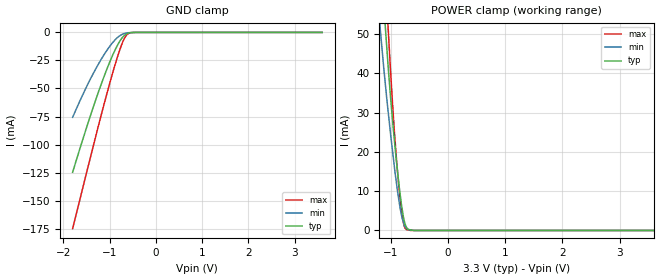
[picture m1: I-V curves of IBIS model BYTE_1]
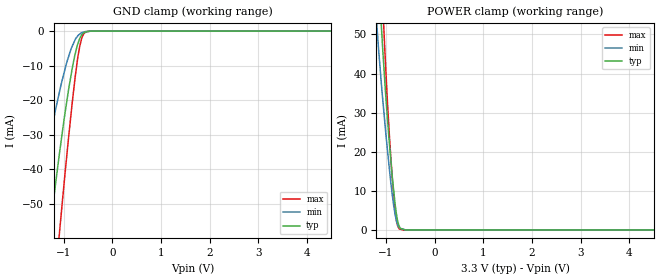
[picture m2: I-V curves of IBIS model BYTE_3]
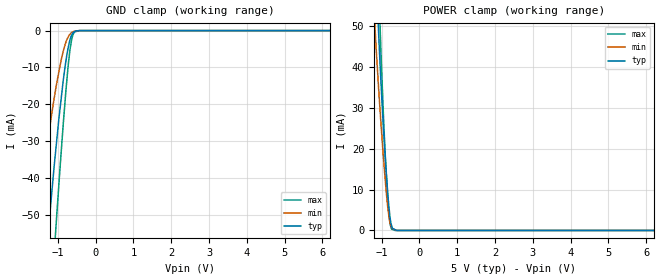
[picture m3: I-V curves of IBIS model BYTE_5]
|Texas Instruments Incorporated
|16-Bit, 250kSPS, Paralell, CMOS, Sampling
|ANALOG-TO-DIGITAL CONVERTERs
| Marketing part#   Digital Voltage Range   Package-type   #pins
|ADS8515IBDBR   1.65 to 5.25   SSOP   28
|ADS8515IBDBRG4   1.65 to 5.25   SSOP   28
|ADS8515IDB   1.65 to 5.25   SSOP   28
|ADS8515IDBG4   1.65 to 5.25   SSOP   28
|ADS8515IDBR   1.65 to 5.25   SSOP   28
|ADS8515IDBRG4   1.65 to 5.25   SSOP   28
[IBIS Ver]   4.0
[File name]   ads8515.ibs
|SIMDE Ver   V2.2 - 201009 - RHL4 - Build 424
[File Rev]   1.0
[Date]   02/09/2011
[Source]   Texas Instruments Incorporated.
   Analog-eLab, HPA
   12500 TI Blvd
   Dallas, TX -75243
   For Support e-mail: elab_ibis@list.ti.com
[Notes]   Revision History:
   1.0: 02/19/2010
   - Initial version of the model
   - Initial Model generated from simulations in TISPICED
   - Model not matched to measurements
   - Model names with a trailing _1 contains the model for
   1.8V [1.65V and 2V].
   - Model names with trailing _3 contains
   the model for 3.3V [3.0V and 3.6V] operation.
   - Model names with trailing _5 contains
   the model for 5V [4.75V and 5.25V] operation.
   - Ignore warnings related to min and max values of ccomp,
   The device process of these products is CMOS. The ccomp
   values are based on PVT variations as seen in simulations
   - Ignore warnings related to typical values not in between
   Min and Max of ccomp for DATA_5 and SYNC_5. These values
   are a mathematical average of the correct buffer high and
   buffer low ccomp value
   - POWER CLAMP and GROUND CLAMP curves differ due to silicon
   topology and hence simulation results
   1.1: 02/09/2011
   - Changed the c_comp order to numerical order instead of the
   order obtained from PVT values.
[Disclaimer]
 This product is designed as an aid for customers of Texas Instruments.
 No warranties, either expressed or implied, with respect to this third
 party software, if any, or with respect to its fitness for any
 particular purpose is claimed by Texas Instruments or the author. The
 software, if any, is provided solely on an "as is" basis. The entire
 risk as to its quality and performance is with the customer
[Copyright] [C] Copyright 2010 Texas Instruments Incorporated.
   All rights reserved.
|   ADS8515
[Component]   ADS8515idb
[Manufacturer] TI
[Package]
| variable   typ   min   max
R_pkg  0.081397   0.036370   0.106720
L_pkg  2.707628nH  1.715680nH  4.109430nH
C_pkg  0.472490pF  0.375470pF  0.646710pF
[Pin] signal_name  model_name  R_pin   L_pin   C_pin
1   VIN   TERM   0.10148  4.01003nH  0.61838pF
2   AGND1   GND   0.09846  3.51545nH  0.60135pF
3   REF   TERM   0.09798  3.16690nH  0.49603pF
4   CAP   TERM   0.04663  2.04507nH  0.43435pF
5   AGND2   GND   0.03637  1.71568nH  0.42202pF
6   D15   DATA   0.06881  1.98435nH  0.38747pF
7   D14   DATA   0.06685  1.93451nH  0.37821pF
8   D13   DATA   0.06409  1.88669nH  0.37548pF
9   D12   DATA   0.06374  1.89612nH  0.38304pF
10   D11   DATA   0.07125  2.05121nH  0.39748pF
11   D10   DATA   0.08925  2.40829nH  0.39818pF
12   D9   DATA   0.09950  3.19736nH  0.49762pF
13   D8   DATA   0.09919  3.53548nH  0.60319pF
14   DGND   GND   0.10221  4.03248nH  0.61888pF
15   D7   DATA   0.10398  4.06578nH  0.61971pF
16   D6   DATA   0.10219  3.59198nH  0.60412pF
17   D5   DATA   0.10129  3.23126nH  0.49728pF
18   D4   DATA   0.08959  2.41469nH  0.39742pF
19   D3   DATA   0.07539  2.12774nH  0.40027pF
20   D2   DATA   0.07005  2.01182nH  0.38846pF
21   D1   DATA   0.06753  1.95025nH  0.37854pF
22   D0   DATA   0.06359  1.87696nH  0.37547pF
23   BYTE   BYTE   0.06489  1.91375nH  0.38429pF
24   R_C   RC   0.07051  2.03154nH  0.39581pF
25   _CS   CS   0.09558  2.51746nH  0.40521pF
26   _BUSY   BUSY   0.10336  3.26890nH  0.49850pF
27   VANA   POWER   0.05864  3.32240nH  0.64671pF
28   VDIG   POWER   0.10672  4.10943nH  0.62626pF
|   Model Selectors
[Model Selector]  BYTE
BYTE_1   1.8V digital Input
BYTE_3   3.3V digital Input
BYTE_5   5V digital Input
[Model Selector]  RC
RC_1   1.8V digital Input
RC_3   3.3V digital Input
RC_5   5V digital Input
[Model Selector]  CS
CS_1   1.8V digital Input
CS_3   3.3V digital Input
CS_5   5V digital Input
[Model Selector]  BUSY
BUSY_1   1.8V digital Output
BUSY_3   3.3V digital Output
BUSY_5   5V digital Output
[Model Selector]  DATA
DATA_1   1.8V digital 3-state
DATA_3   3.3V digital 3-state
DATA_5   5V digital 3-state
[Model Selector] TERM
TERM_1   1.8V nominal termination
TERM_3   3.3V nominal termination
TERM_5   5.0V nominal termination
|   TERM_1
[Model]  TERM_1
Model_type Terminator
C_comp   1.0e-20F  1.0e-20F  1.0e-20F
|   typ   min   max
[Voltage Range]   1.8V   1.71V   1.89V
[POWER Clamp Reference]   1.8V   1.71V   1.89V
[GND Clamp Reference]   0V   0V   0V
|Ambient Temperature   25   85   -40
|Junction Temperature
[Temperature Range]   32   92   -40
|   TERM_3
[Model]  TERM_3
Model_type Terminator
C_comp   1.0e-20F  1.0e-20F  1.0e-20F
|   typ   min   max
[Voltage Range]   3.3V   3.0V   3.6V
[POWER Clamp Reference]   3.3V   3.0V   3.6V
[GND Clamp Reference]   0V   0V   0V
|Ambient Temperature   25   85   -40
|Junction Temperature
[Temperature Range]   32   92   -40
|   TERM_5
[Model]  TERM_5
Model_type Terminator
C_comp   1.0e-20F  1.0e-20F  1.0e-20F
|   typ   min   max
[Voltage Range]   5.0V   4.75V   5.25V
[POWER Clamp Reference]   5.0V   4.75V   5.25V
[GND Clamp Reference]   0V   0V   0V
|Ambient Temperature   25   85   -40
|Junction Temperature
[Temperature Range]   32   92   -40
| Models and submodels in the file (18): BYTE_1 (Input), BYTE_3 (Input), BYTE_5 (Input), RC_1 (Input), RC_3 (Input), RC_5 (Input), CS_1 (Input), CS_3 (Input), CS_5 (Input), BUSY_1 (Output), BUSY_3 (Output), BUSY_5 (Output), DATA_1 (3-state), DATA_3 (3-state), DATA_5 (3-state), TERM_1 (Terminator), TERM_3 (Terminator), TERM_5 (Terminator)
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|   BYTE INPUT Model  1.8V
[Model] BYTE_1
Model_type Input
Vinl = 0.8
Vinh = 1.08
|   typ   min   max
C_comp   7.6429900e-12   6.7918740e-12  8.3793010e-12
| variable   typ   min   max
[Voltage Range]   3.3V   2.0V   5.5V
[POWER Clamp Reference]  3.3V   2.0V   5.5V
[GND Clamp Reference]   0.0V   0.0V   0.0V
|Operating Temperature
[Temperature Range]   27   85   -40
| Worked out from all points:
|   GND clamp passes 1 mA (typ) near -0.62 V on its own axis
|   POWER clamp passes 1 mA (typ) near -0.73 V on its own axis
[GND Clamp]
|   Voltage   I  typ   I  min   I  max
-1.8V     -124.7mA   -75.71mA   -174.9mA
-1.614V   -99.82mA   -58.49mA   -144.1mA
-1.376V   -69.35mA   -38.38mA   -105mA
-1.231V   -51.83mA   -27.37mA   -81.45mA
-1.059V   -32.69mA   -16.02mA   -54.6mA
-933.2mV  -20.21mA   -9.063mA   -35.98mA
-789.8mV  -8.518mA   -3.242mA   -16.72mA
-708.6mV  -3.828mA   -1.413mA   -7.743mA
-672.9mV  -2.354mA   -890.4uA   -4.758mA
-610.4mV  -794.8uA   -377.7uA   -1.488mA
-434.6mV  -9.5uA     -9.497uA   -8.839uA
3.595V    0A         0A         0A
[POWER Clamp]
|   Voltage   I  typ   I  min   I  max
-1.8V     224.9mA    179.5mA    278.6mA
-1.183V   71.28mA    51.11mA    90.16mA
-1.092V   51.02mA    36.78mA    64.11mA
-1.044V   41.4mA     30.05mA    51.07mA
-970mV    28.2mA     20.28mA    32.38mA
-937.8mV  23.1mA     16.26mA    25.33mA
-861.7mV  12.28mA    8.001mA    11.54mA
-796.2mV  4.976mA    2.872mA    3.167mA
-764.9mV  2.476mA    1.409mA    1.097mA
-728.4mV  890.3uA    554.4uA    223.6uA
-604.5mV  9.09uA     23.83uA    5.645uA
3.595V    0A         0A         0A
|   BYTE INPUT Model  3.3V
[Model] BYTE_3
Model_type Input
Vinl = 0.8
Vinh = 2.16
|   typ   min   max
C_comp   6.5925360e-12  5.8425430e-12   7.3059290e-12
[Voltage Range]   3.3   3   3.6
[Temperature Range]   27   85   -40
[Power Clamp Reference]   3.3   3   3.6
[GND Clamp Reference]   0   0   0
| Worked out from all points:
|   GND clamp passes 1 mA (typ) near -0.62 V on its own axis
|   POWER clamp passes 1 mA (typ) near -0.73 V on its own axis
[GND Clamp]
|   Voltage   I  typ   I  min   I  max
-3.3V     -336.7mA   -238mA     -424.2mA
-1.607V   -98.95mA   -57.98mA   -143mA
-1.291V   -58.99mA   -31.77mA   -91.17mA
-1.093V   -36.36mA   -18.22mA   -59.88mA
-1.068V   -33.75mA   -16.61mA   -55.98mA
-935.3mV  -20.51mA   -9.123mA   -36.31mA
-814.5mV  -10.22mA   -4.148mA   -19.82mA
-712.1mV  -3.937mA   -1.474mA   -8.079mA
-626.8mV  -1.072mA   -454.8uA   -2.11mA
-557.5mV  -326.6uA   -151.8uA   -403.9uA
-433.6mV  -11.6uA    -11.54uA   -8.503uA
6.59V     0A         0A         0A
[POWER Clamp]
|   Voltage   I  typ   I  min   I  max
-3.3V     615.9mA    518.7mA    751mA
-1.199V   74.96mA    54mA       94.9mA
-1.158V   65.6mA     46.9mA     82.83mA
-1.094V   51.69mA    37.06mA    64.81mA
-1.065V   45.36mA    32.88mA    56.55mA
-1.025V   37.84mA    27.49mA    45.98mA
-966mV    27.59mA    19.83mA    31.46mA
-872.4mV  13.62mA    8.955mA    13.24mA
-807.6mV  5.944mA    3.544mA    4.277mA
-734.2mV  1.045mA    676.8uA    292uA
-604.8mV  9.134uA    29.43uA    5.753uA
6.59V     0A         0A         0A
|   BYTE INPUT Model  5V
[Model] BYTE_5
Model_type Input
Vinl = 0.8
Vinh = 3.25
|   typ   min   max
C_comp   5.8288830e-12   5.2095660e-12   6.4082030e-12
[Voltage Range]   5   4.75   5.25
[Temperature Range]   27   85   -40
[Power Clamp Reference]   5   4.75   5.25
[GND Clamp Reference]   0   0   0
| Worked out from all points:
|   GND clamp passes 1 mA (typ) near -0.62 V on its own axis
|   POWER clamp passes 1 mA (typ) near -0.73 V on its own axis
[GND Clamp]
|   Voltage   I  typ   I  min   I  max
-5V       -582.7mA   -439.8mA   -706.6mA
-1.699V   -111.1mA   -66.3mA    -158.2mA
-1.544V   -90.71mA   -52.39mA   -132.6mA
-1.25V    -54.12mA   -28.91mA   -84.52mA
-1.09V    -35.96mA   -17.92mA   -59.34mA
-1.046V   -31.44mA   -15.18mA   -52.55mA
-865.2mV  -14.22mA   -5.966mA   -26.47mA
-728.2mV  -4.723mA   -1.772mA   -9.676mA
-680.2mV  -2.579mA   -1.009mA   -5.304mA
-634.6mV  -1.246mA   -510.3uA   -2.454mA
-560.7mV  -292.9uA   -156uA     -482.7uA
9.985V    0A         0A         0A
[POWER Clamp]
|   Voltage   I  typ   I  min   I  max
-5V       1.064A     908.8mA    1.291A
-1.172V   68.87mA    49.36mA    86.94mA
-1.084V   49.64mA    35.71mA    61.98mA
-1.053V   43.05mA    31.16mA    53.52mA
-1.016V   36.14mA    26.07mA    43.48mA
-956.5mV  25.94mA    18.5mA     29.33mA
-907.6mV  18.53mA    12.89mA    19.4mA
-814.2mV  6.662mA    4.011mA    5.005mA
-782.5mV  3.72mA     2.12mA     2.075mA
-751.7mV  1.739mA    1.217mA    789.7uA
-646mV    214.3uA    184.7uA    4.043uA
9.985V    0A         0A         0A
